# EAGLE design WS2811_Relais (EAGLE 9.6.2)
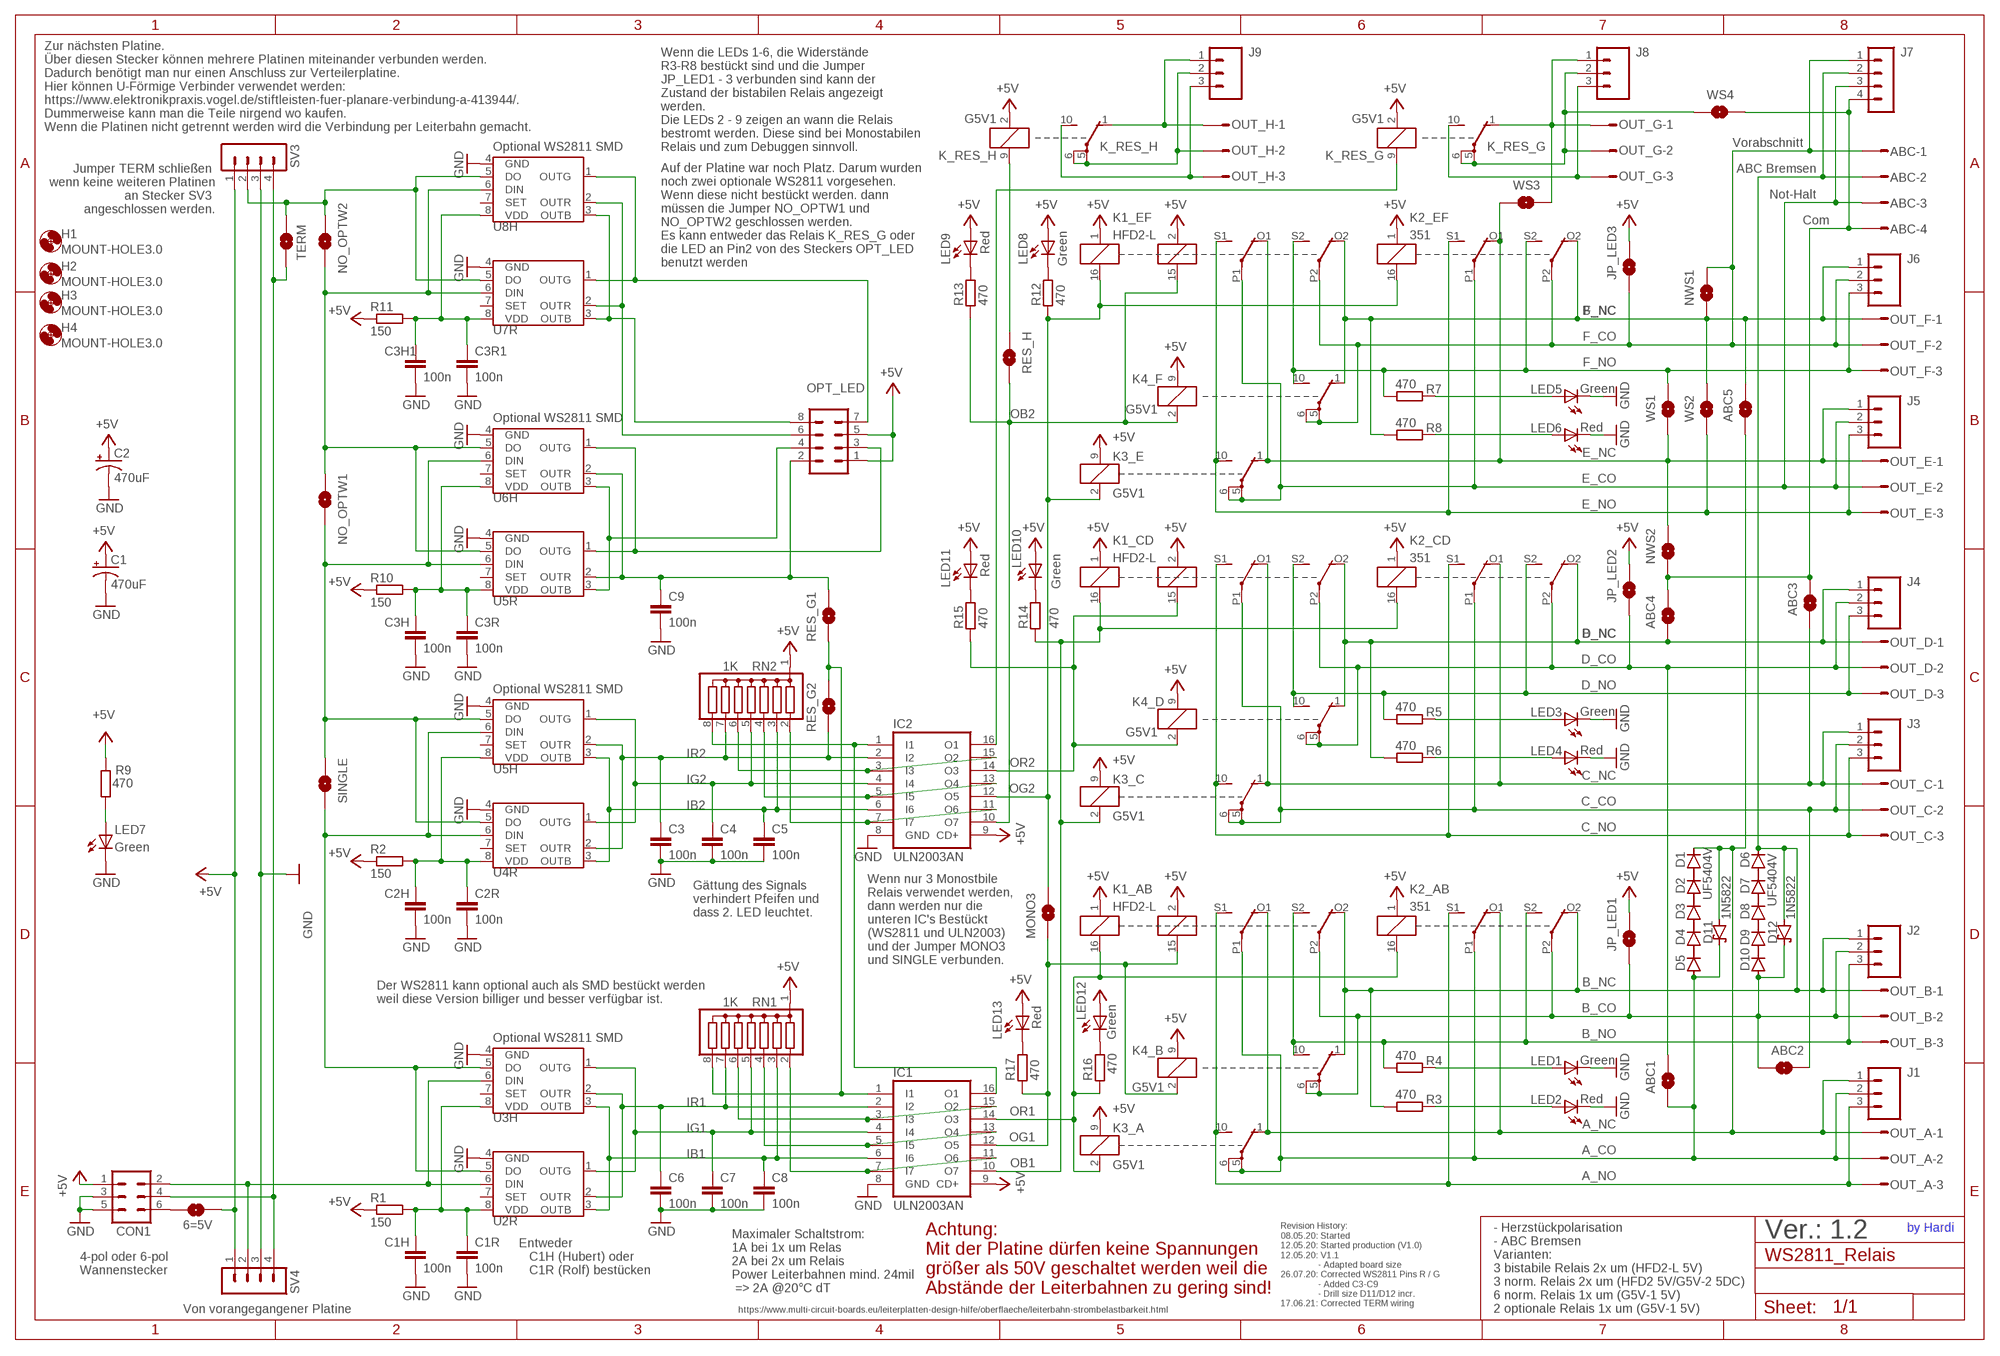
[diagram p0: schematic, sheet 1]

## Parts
6=5V  SOLDERJUMPERNO  [SJ_2S-NO]
ABC  STL1550-4ON_BOARD  [STL1550-4_ON_BOARD]
ABC1  SOLDERJUMPERNO  [SJ_2S-NO]
ABC2  SOLDERJUMPERNO  [SJ_2S-NO]
ABC3  SOLDERJUMPERNO  [SJ_2S-NO]
ABC4  SOLDERJUMPERNO  [SJ_2S-NO]
ABC5  SOLDERJUMPERNO  [SJ_2S-NO]
C1  470uF  SPARKFUN-CAPACITORS_100UF-25V-20%(PTH)  [SPARKFUN-CAPACITORS_CPOL-RADIAL-100UF-25V]
C1H  100n  C-EUC1206  [C1206]
C1R  100n  C-EU025-024X044  [C025-024X044]
C2  470uF  SPARKFUN-CAPACITORS_100UF-25V-20%(PTH)  [SPARKFUN-CAPACITORS_CPOL-RADIAL-100UF-25V]
C2H  100n  C-EUC1206  [C1206]
C2R  100n  C-EU025-024X044  [C025-024X044]
C3  100n  C-EU025-024X044  [C025-024X044]
C3H  100n  C-EUC1206  [C1206]
C3H1  100n  C-EUC1206  [C1206]
C3R  100n  C-EU025-024X044  [C025-024X044]
C3R1  100n  C-EU025-024X044  [C025-024X044]
C4  100n  C-EU025-024X044  [C025-024X044]
C5  100n  C-EU025-024X044  [C025-024X044]
C6  100n  C-EU025-024X044  [C025-024X044]
C7  100n  C-EU025-024X044  [C025-024X044]
C8  100n  C-EU025-024X044  [C025-024X044]
C9  100n  C-EU025-024X044  [C025-024X044]
CON1  ML6  [ML6]
D1  UF5404V  [DO201-15-V]
D2  UF5404V  [DO201-15-V]
D3  UF5404V  [DO201-15-V]
D4  UF5404V  [DO201-15-V]
D5  UF5404V  [DO201-15-V]
D6  UF5404V  [DO201-15-V]
D7  UF5404V  [DO201-15-V]
D8  UF5404V  [DO201-15-V]
D9  UF5404V  [DO201-15-V]
D10  UF5404V  [DO201-15-V]
D11  1N5822  [DO41-7.6]
D12  1N5822  [DO41-7.6]
H1  MOUNT-HOLE3.0  [3,0]
H2  MOUNT-HOLE3.0  [3,0]
H3  MOUNT-HOLE3.0  [3,0]
H4  MOUNT-HOLE3.0  [3,0]
IC1  ULN2003AN  [DIL16]
IC2  ULN2003AN  [DIL16]
J1  M03PTH  [1X03]
J2  M03PTH  [1X03]
J3  M03PTH  [1X03]
J4  M03PTH  [1X03]
J5  M03PTH  [1X03]
J6  M03PTH  [1X03]
J7  MA04-1  [MA04-1]
J8  M03PTH  [1X03]
J9  M03PTH  [1X03]
JP_LED1  SOLDERJUMPERNO  [SJ_2S-NO]
JP_LED2  SOLDERJUMPERNO  [SJ_2S-NO]
JP_LED3  SOLDERJUMPERNO  [SJ_2S-NO]
K1_AB  HFD2-L  [HFD2-L]
K1_CD  HFD2-L  [HFD2-L]
K1_EF  HFD2-L  [HFD2-L]
K2_AB  351  [351]
K2_CD  351  [351]
K2_EF  351  [351]
K3_A  G5V1  [G5V1]
K3_C  G5V1  [G5V1]
K3_E  G5V1  [G5V1]
K4_B  G5V1  [G5V1]
K4_D  G5V1  [G5V1]
K4_F  G5V1  [G5V1]
K_RES_G  G5V1  [G5V1]
K_RES_H  G5V1  [G5V1]
LED1  Green  LED3MM  [LED3MM]
LED2  Red  LED3MM  [LED3MM]
LED3  Green  LED3MM  [LED3MM]
LED4  Red  LED3MM  [LED3MM]
LED5  Green  LED3MM  [LED3MM]
LED6  Red  LED3MM  [LED3MM]
LED7  Green  LED3MM  [LED3MM]
LED8  Green  LED3MM  [LED3MM]
LED9  Red  LED3MM  [LED3MM]
LED10  Green  LED3MM  [LED3MM]
LED11  Red  LED3MM  [LED3MM]
LED12  Green  LED3MM  [LED3MM]
LED13  Red  LED3MM  [LED3MM]
MONO3  SOLDERJUMPERNO  [SJ_2S-NO]
NO_OPTW1  SOLDERJUMPERNO  [SJ_2S-NO]
NO_OPTW2  SOLDERJUMPERNO  [SJ_2S-NO]
NWS1  SOLDERJUMPERNO  [SJ_2S-NO]
NWS2  SOLDERJUMPERNO  [SJ_2S-NO]
OPT_LED  CON-HARTING-ML_ML08  [CON-HARTING-ML_ML08]
OUT_A  STL1550-3  [STL1550-3]
OUT_B  STL1550-3  [STL1550-3]
OUT_C  STL1550-3  [STL1550-3]
OUT_D  STL1550-3  [STL1550-3]
OUT_E  STL1550-3  [STL1550-3]
OUT_F  STL1550-3  [STL1550-3]
OUT_G  STL1550-3  [STL1550-3]
OUT_H  STL1550-3  [STL1550-3]
R1  150  RCL_R-EU_0207/2V  [RCL_0207/2V]
R2  150  RCL_R-EU_0207/2V  [RCL_0207/2V]
R3  470  R0204/2V  [0204/2V]
R4  470  R0204/2V  [0204/2V]
R5  470  R0204/2V  [0204/2V]
R6  470  R0204/2V  [0204/2V]
R7  470  R0204/2V  [0204/2V]
R8  470  R0204/2V  [0204/2V]
R9  470  R0204/2V  [0204/2V]
R10  150  RCL_R-EU_0207/2V  [RCL_0207/2V]
R11  150  RCL_R-EU_0207/2V  [RCL_0207/2V]
R12  470  R0204/2V  [0204/2V]
R13  470  R0204/2V  [0204/2V]
R14  470  R0204/2V  [0204/2V]
R15  470  R0204/2V  [0204/2V]
R16  470  R0204/2V  [0204/2V]
R17  470  R0204/2V  [0204/2V]
RES_G1  SOLDERJUMPERNO  [SJ_2S-NO]
RES_G2  SOLDERJUMPERNO  [SJ_2S-NO]
RES_H  SOLDERJUMPERNO  [SJ_2S-NO]
RN1  1K  G07R  [SIL8]
RN2  1K  G07R  [SIL8]
SINGLE  SOLDERJUMPERNO  [SJ_2S-NO]
SV3  MA04-1  [MA04-1]
SV4  MA04-1  [MA04-1]
TERM  SOLDERJUMPERNO  [SJ_2S-NO]
U2R  TINY45-20-DIP  S3PO_MODUL_WS2811_SOUND_MP3-TF-16P_WS2811_AND_ATTINY_WS2811-ICTINY45-20-DIP  [S3PO_MODUL_WS2811_SOUND_MP3-TF-16P_WS2811_AND_ATTINY_WS2811_DIP08]
U3H  WS2811 SOT-8  S3PO_MODUL_WS2811_SOUND_MP3-TF-16P_WS2811_AND_ATTINY_WS2811-ICSOP8  [SOP8]
U4R  TINY45-20-DIP  S3PO_MODUL_WS2811_SOUND_MP3-TF-16P_WS2811_AND_ATTINY_WS2811-ICTINY45-20-DIP  [S3PO_MODUL_WS2811_SOUND_MP3-TF-16P_WS2811_AND_ATTINY_WS2811_DIP08]
U5H  WS2811 SOT-8  S3PO_MODUL_WS2811_SOUND_MP3-TF-16P_WS2811_AND_ATTINY_WS2811-ICSOP8  [SOP8]
U5R  TINY45-20-DIP  S3PO_MODUL_WS2811_SOUND_MP3-TF-16P_WS2811_AND_ATTINY_WS2811-ICTINY45-20-DIP  [S3PO_MODUL_WS2811_SOUND_MP3-TF-16P_WS2811_AND_ATTINY_WS2811_DIP08]
U6H  WS2811 SOT-8  S3PO_MODUL_WS2811_SOUND_MP3-TF-16P_WS2811_AND_ATTINY_WS2811-ICSOP8  [SOP8]
U7R  TINY45-20-DIP  S3PO_MODUL_WS2811_SOUND_MP3-TF-16P_WS2811_AND_ATTINY_WS2811-ICTINY45-20-DIP  [S3PO_MODUL_WS2811_SOUND_MP3-TF-16P_WS2811_AND_ATTINY_WS2811_DIP08]
U8H  WS2811 SOT-8  S3PO_MODUL_WS2811_SOUND_MP3-TF-16P_WS2811_AND_ATTINY_WS2811-ICSOP8  [SOP8]
WS1  SOLDERJUMPERNO  [SJ_2S-NO]
WS2  SOLDERJUMPERNO  [SJ_2S-NO]
WS3  SOLDERJUMPERNO  [SJ_2S-NO]
WS4  SOLDERJUMPERNO  [SJ_2S-NO]

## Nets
+5V: 6=5V.2 C1.1(+) C2.1(+) CON1.1 IC1.9(CD+) IC2.9(CD+) JP_LED1.2 JP_LED2.2 JP_LED3.2 K1_AB.1 K1_AB.2 K1_CD.1 K1_CD.2 K1_EF.1 K1_EF.2 K2_AB.1 K2_CD.1 K2_EF.1 K3_A.9 K3_C.9 K3_E.9 K4_B.9 K4_D.9 K4_F.9 K_RES_G.2 K_RES_H.2 LED8.A LED9.A LED10.A LED11.A LED12.A LED13.A OPT_LED.1 OPT_LED.5 R1.1 R2.1 R9.1 R10.1 R11.1 RN1.1 RN2.1 SV3.1 SV4.1
A_CO: ABC1.1 D5.A D11.C J1.2 K1_AB.P1(2:P) K2_AB.P1(2:P) K3_A.5(2:P) K3_A.6(2:P) OUT_A.2
A_NC: ABC5.2 D1.C D11.A J1.1 K1_AB.O1(2:O) K2_AB.O1(2:O) K3_A.1(2:O) OUT_A.1
A_NO: J1.3 K1_AB.S1(2:S) K2_AB.S1(2:S) K3_A.10(2:S) OUT_A.3
B_CO: ABC2.1 D10.A D12.C J2.2 JP_LED1.1 K1_AB.P2(3:P) K2_AB.P2(3:P) K4_B.5(2:P) K4_B.6(2:P) OUT_B.2
B_NC: ABC.2 D6.C D12.A J2.1 J7.2 K1_AB.O2(3:O) K2_AB.O2(3:O) K4_B.1(2:O) OUT_B.1 R3.2
B_NO: J2.3 K1_AB.S2(3:S) K2_AB.S2(3:S) K4_B.10(2:S) OUT_B.3 R4.2
C_CO: ABC2.2 J3.2 K1_CD.P1(2:P) K2_CD.P1(2:P) K3_C.5(2:P) K3_C.6(2:P) OUT_C.2
C_NC: ABC3.2 J3.1 K1_CD.O1(2:O) K2_CD.O1(2:O) K3_C.1(2:O) OUT_C.1
C_NO: J3.3 K1_CD.S1(2:S) K2_CD.S1(2:S) K3_C.10(2:S) OUT_C.3
COM: ABC3.1 ABC4.1 ABC.4 J7.4 NWS2.2 WS4.1
CTRL_H_OB2: K_RES_H.9 RES_H.2
D_CO: ABC1.2 J4.2 JP_LED2.1 K1_CD.P2(3:P) K2_CD.P2(3:P) K4_D.5(2:P) K4_D.6(2:P) OUT_D.2
D_NC: ABC4.2 J4.1 K1_CD.O2(3:O) K2_CD.O2(3:O) K4_D.1(2:O) OUT_D.1 R6.2
D_NO: J4.3 K1_CD.S2(3:S) K2_CD.S2(3:S) K4_D.10(2:S) OUT_D.3 R5.2
DI_WS1: CON1.2 SV4.2 U2R.6(DIN) U3H.6(DIN)
DO1_DI2: SINGLE.2 U2R.5(DO) U3H.5(DO) U4R.6(DIN) U5H.6(DIN)
DO2_DI3: NO_OPTW1.2 SINGLE.1 U4R.5(DO) U5H.5(DO) U5R.6(DIN) U6H.6(DIN)
DO3_DI4: NO_OPTW1.1 NO_OPTW2.2 U5R.5(DO) U6H.5(DO) U7R.6(DIN) U8H.6(DIN)
DO4_NEXT_TERM: NO_OPTW2.1 SV3.2 TERM.2 U7R.5(DO) U8H.5(DO)
DO_RETURN: CON1.4 SV3.4 SV4.4 TERM.1
E_CO: ABC.3 J5.2 J7.3 K1_EF.P1(2:P) K2_EF.P1(2:P) K3_E.5(2:P) K3_E.6(2:P) OUT_E.2
E_NC: J5.1 K1_EF.O1(2:O) K2_EF.O1(2:O) K3_E.1(2:O) NWS2.1 OUT_E.1 WS1.2 WS3.2
E_NO: J5.3 K1_EF.S1(2:S) K2_EF.S1(2:S) K3_E.10(2:S) OUT_E.3 WS2.2
F_CO: ABC.1 J6.2 J7.1 JP_LED3.1 K1_EF.P2(3:P) K2_EF.P2(3:P) K4_F.5(2:P) K4_F.6(2:P) NWS1.1 OUT_F.2
F_NC: ABC5.1 J6.1 K1_EF.O2(3:O) K2_EF.O2(3:O) K4_F.1(2:O) NWS1.2 OUT_F.1 R8.2 WS2.1
F_NO: J6.3 K1_EF.S2(3:S) K2_EF.S2(3:S) K4_F.10(2:S) OUT_F.3 R7.2 WS1.1
G_COM: J8.2 K_RES_G.5(2:P) K_RES_G.6(2:P) OUT_G.2 WS4.2
G_NC: J8.1 K_RES_G.1(2:O) OUT_G.1 WS3.1
G_NO: J8.3 K_RES_G.10(2:S) OUT_G.3
GND: C1.2(-) C1H.2 C1R.2 C2.2(-) C2H.2 C2R.2 C3.2 C3H1.2 C3H.2 C3R1.2 C3R.2 C4.2 C5.2 C6.2 C7.2 C8.2 C9.2 CON1.3 CON1.5 IC1.8(GND) IC2.8(GND) LED1.K(C) LED2.K(C) LED3.K(C) LED4.K(C) LED5.K(C) LED6.K(C) LED7.K(C) SV3.3 SV4.3 U2R.4(GND) U3H.4(GND) U4R.4(GND) U5H.4(GND) U5R.4(GND) U6H.4(GND) U7R.4(GND) U8H.4(GND)
H_COM: J9.2 K_RES_H.5(2:P) K_RES_H.6(2:P) OUT_H.2
H_NC: J9.1 K_RES_H.1(2:O) OUT_H.1
H_NO: J9.3 K_RES_H.10(2:S) OUT_H.3
IB1: C8.1 IC1.6(I6) RN1.3 U2R.3(OUTB) U3H.3(OUTB)
IB1_2: IC1.7(I7) IC1.11(O6) RN1.2
IB2: C5.1 IC2.6(I6) RN2.3 U4R.3(OUTB) U5H.3(OUTB)
IB2_2: IC2.7(I7) IC2.11(O6) RN2.2
IB3: OPT_LED.4 U5R.3(OUTB) U6H.3(OUTB)
IB4: OPT_LED.8 U7R.3(OUTB) U8H.3(OUTB)
IG1: C7.1 IC1.4(I4) RN1.5 U2R.1(OUTG) U3H.1(OUTG)
IG1_2: IC1.5(I5) IC1.13(O4) RN1.4
IG2: C4.1 IC2.4(I4) RN2.5 U4R.1(OUTG) U5H.1(OUTG)
IG2_2: IC2.5(I5) IC2.13(O4) RN2.4
IG3: OPT_LED.3 U5R.1(OUTG) U6H.1(OUTG)
IG4: OPT_LED.7 U7R.1(OUTG) U8H.1(OUTG)
IR1: C6.1 IC1.2(I2) RN1.7 U2R.2(OUTR) U3H.2(OUTR)
IR1_2: IC1.3(I3) IC1.15(O2) RN1.6
IR2: C3.1 IC2.2(I2) RES_G2.2 RN2.7 U4R.2(OUTR) U5H.2(OUTR)
IR2_2: IC2.3(I3) IC2.15(O2) RN2.6
IR3: IC1.1(I1) RES_G1.2 RES_G2.1 RN1.8
IR3_2: C9.1 OPT_LED.2 RES_G1.1 U5R.2(OUTR) U6H.2(OUTR)
IR3_3: IC1.16(O1) IC2.1(I1) RN2.8
IR4: OPT_LED.6 U7R.2(OUTR) U8H.2(OUTR)
LED2: LED2.A R3.1
LED3: LED3.A R5.1
LED4: LED4.A R6.1
LED_1: LED1.A R4.1
LED_5: LED5.A R7.1
LED_6: LED6.A R8.1
LED_7: LED7.A R9.2
N$6: 6=5V.1 CON1.6
N$16: D1.A D2.C
N$19: D2.A D3.C
N$21: D3.A D4.C
N$23: D4.A D5.C
N$24: D7.A D8.C
N$25: D8.A D9.C
N$26: D9.A D10.C
N$27: D6.A D7.C
N$42: LED8.K(C) R12.1
N$43: LED9.K(C) R13.1
N$44: LED10.K(C) R14.1
N$45: LED11.K(C) R15.1
N$46: LED12.K(C) R16.1
N$47: LED13.K(C) R17.1
OB1: IC1.10(O7) K1_CD.16 K2_CD.16 K3_C.2 R14.2
OB2: IC2.10(O7) K1_EF.15 K4_F.2 R13.2 RES_H.1
OG1: IC1.12(O5) K1_AB.15 K4_B.2 MONO3.2 R17.2
OG2: IC2.12(O5) K1_EF.16 K2_EF.16 K3_E.2 MONO3.1 R12.2
OR1: IC1.14(O3) K1_AB.16 K2_AB.16 K3_A.2 R16.2
OR2: IC2.14(O3) K1_CD.15 K4_D.2 R15.2
OR3: IC2.16(O1) K_RES_G.9
PWR_WS1: C1H.1 C1R.1 R1.2 U2R.8(VDD) U3H.8(VDD)
PWR_WS2: C2H.1 C2R.1 R2.2 U4R.8(VDD) U5H.8(VDD)
PWR_WS3: C3H.1 C3R.1 R10.2 U5R.8(VDD) U6H.8(VDD)
PWR_WS4: C3H1.1 C3R1.1 R11.2 U7R.8(VDD) U8H.8(VDD)
Unconnected: U2R.7(SET) U3H.7(SET) U4R.7(SET) U5H.7(SET) U5R.7(SET) U6H.7(SET) U7R.7(SET) U8H.7(SET)

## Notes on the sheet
- Wenn die LEDs 1-6, die Widerstände
  R3-R8 bestückt sind und die Jumper 
  JP_LED1 - 3 verbunden sind kann der 
  Zustand der bistabilen Relais angezeigt
  werden. 
  Die LEDs 2 - 9 zeigen an wann die Relais
  bestromt werden. Diese sind bei Monostabilen
  Relais und zum Debuggen sinnvoll.
- Zur nächsten Platine. 
  Über diesen Stecker können mehrere Platinen miteinander verbunden werden.
  Dadurch benötigt man nur einen Anschluss zur Verteilerplatine.
  Hier können U-Förmige Verbinder verwendet werden: 
  https://www.elektronikpraxis.vogel.de/stiftleisten-fuer-planare-verbindung-a-413944/.
  Dummerweise kann man die Teile nirgend wo kaufen.
  Wenn die Platinen nicht getrennt werden wird die Verbindung per Leiterbahn gemacht.
- Vorabschnitt
- Optional WS2811 SMD
- Jumper TERM schließen 
  wenn keine weiteren Platinen
  an Stecker SV3 
  angeschlossen werden.
- ABC Bremsen
- Not-Halt
- Com
- Auf der Platine war noch Platz. Darum wurden
  noch zwei optionale WS2811 vorgesehen. 
  Wenn diese nicht bestückt werden. dann 
  müssen die Jumper NO_OPTW1 und 
  NO_OPTW2 geschlossen werden. 
  Es kann entweder das Relais K_RES_G oder 
  die LED an Pin2 von des Steckers OPT_LED 
  benutzt werden
- Optional WS2811 SMD
- Optional WS2811 SMD
- Gättung des Signals
  verhindert Pfeifen und
  dass 2. LED leuchtet.
- Wenn nur 3 Monostbile
  Relais verwendet werden,
  dann werden nur die
  unteren IC's Bestückt
  (WS2811 und ULN2003)
  und der Jumper MONO3
  und SINGLE verbunden.
- Der WS2811 kann optional auch als SMD bestückt werden
  weil diese Version billiger und besser verfügbar ist.
- Optional WS2811 SMD
- Ver.: 1.2
- Achtung:
  Mit der Platine dürfen keine Spannungen
  größer als 50V geschaltet werden weil die
  Abstände der Leiterbahnen zu gering sind!
- Revision History:
  08.05.20: Started
  12.05.20: Started production (V1.0)
  12.05.20: V1.1
                 - Adapted board size
  26.07.20: Corrected WS2811 Pins R / G
                 - Added C3-C9
                 - Drill size D11/D12 incr.
  17.06.21: Corrected TERM wiring
- - Herzstückpolarisation
  - ABC Bremsen
  Varianten:
  3 bistabile Relais 2x um (HFD2-L 5V)
  3 norm. Relais 2x um (HFD2 5V/G5V-2 5DC)
  6 norm. Relais 1x um (G5V-1 5V)
  2 optionale Relais 1x um (G5V-1 5V)
- by Hardi
- Maximaler Schaltstrom:
  1A bei 1x um Relas
  2A bei 2x um Relais
  Power Leiterbahnen mind. 24mil
   => 2A @20°C dT
- 4-pol oder 6-pol 
  Wannenstecker
- Entweder 
     C1H (Hubert) oder 
     C1R (Rolf) bestücken
- https://www.multi-circuit-boards.eu/leiterplatten-design-hilfe/oberflaeche/leiterbahn-strombelastbarkeit.html
- Von vorangegangener Platine

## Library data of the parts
6=5V ABC1-ABC5 JP_LED1-JP_LED3 MONO3 NO_OPTW1 NO_OPTW2 NWS1 NWS2 RES_G1 RES_G2 RES_H SINGLE TERM WS1-WS4 = SparkFun-Retired:SOLDERJUMPER: Solder Jumper
ABC = SchraubStecker3.5:STL1550-4: CONNECTOR Rastermass 3.5 mm Kabel: AK(Z)1550 Platine: STL(Z)1550 Ali: KF2EDG-3.5
C1 C2 = Sound_MP3-TF-16P_and_WS2811:SPARKFUN-CAPACITORS_100UF-25V-20%(PTH): CAP-08439; PROD_ID: CAP-08439
C1H C1R C2H C2R C3 C3H C3H1 C3R C3R1 C4-C9 = rcl:C-EU: CAPACITOR, European symbol; SPICEPREFIX: C
CON1 = con-harting-ml:ML6: HARTING; OC_FARNELL: unknown; OC_NEWARK: unknown
D1-D10 = diode:UF5404: DIODE
D11 D12 = diode:1N5822: 1.0A SCHOTTKY BARRIER RECTIFIER
H1-H4 = holes:MOUNT-HOLE: MOUNTING HOLE with drill center marker
IC1 IC2 = uln-udn:ULN2003A: DRIVER ARRAY; REICHELT: ULN 2003A STM; REICHELT_EU: 0,22 €; REICHELT_LNK: https://www.reichelt.de/seven-darlington-arrays-dip-16-uln-2003a-stm-p216685.html?&trstct=pos_0
J1-J6 J8 J9 = SparkFun-Connectors:M03: Header 3 Standard 3-pin 0.1" header. Use with straight break away headers (SKU : PRT-00116), right angle break away headers (PRT-00553), swiss pins (PRT-00743), machine pins (PRT-00117), and female headers (PRT-00115). Molex polarized connector foot print use with SKU : PRT-08232 with associated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
J7 SV3 SV4 = con-lstb:MA04-1: PIN HEADER
K1_AB K1_CD K1_EF = WS2811_Relais:HFD2-L: RELAY 2 x switch, HFD2-L by Hardi; OC_FARNELL: unknown; OC_NEWARK: unknown
K2_AB K2_CD K2_EF = relay:351: RELAY 2 x switch, Omron; OC_FARNELL: unknown; OC_NEWARK: unknown
K3_A K3_C K3_E K4_B K4_D K4_F K_RES_G K_RES_H = relay:G5V1: RELAY 1 x switch, 0.5 A/125 V AC, 1 A/24 V DC , Omron; MPN: G5V-1-DC24; OC_FARNELL: 9949593; OC_NEWARK: 36M6377
LED1-LED13 = Arduino_fuer_LEDs_DCC_2:LED: LED
OPT_LED = PushButtonAction_4017_2:CON-HARTING-ML_ML08: Modified by Hardi; OC_FARNELL: unknown; OC_NEWARK: unknown
OUT_A OUT_B OUT_C OUT_D OUT_E OUT_F OUT_G OUT_H = SchraubStecker3.5:STL1550-3: CONNECTOR Rastermass 3.5 mm Kabel: AK(Z)1550 Platine: STL(Z)1550 Ali: KF2EDG-3.5
R1 R2 R10 R11 = Sound_MP3-TF-16P_and_WS2811:RCL_R-EU_: RESISTOR, European symbol; SPICEPREFIX: R
R3-R9 R12-R17 = Arduino_fuer_LEDs_DCC_2:R: RESISTOR, European symbol
RN1 RN2 = resistor-sil:G07R: SIL RESISTOR; OC_FARNELL: unknown; OC_NEWARK: unknown
U2R U4R U5R U7R = S3PO_Modul_WS2811:S3PO_MODUL_WS2811_SOUND_MP3-TF-16P_WS2811_AND_ATTINY_WS2811-IC: Die Pin Nummern für R und G sind getauscht damit sie gleich angesteuert werden wie die WS2812. Der Daten Strom der WS2811 ist RGB, Beim WS2812 ist es aber GRB.; PROD_ID: IC-09439
U3H U5H U6H U8H = S3PO_Modul_WS2811:S3PO_MODUL_WS2811_SOUND_MP3-TF-16P_WS2811_AND_ATTINY_WS2811-IC: Die Pin Nummern für R und G sind getauscht damit sie gleich angesteuert werden wie die WS2812. Der Daten Strom der WS2811 ist RGB, Beim WS2812 ist es aber GRB.

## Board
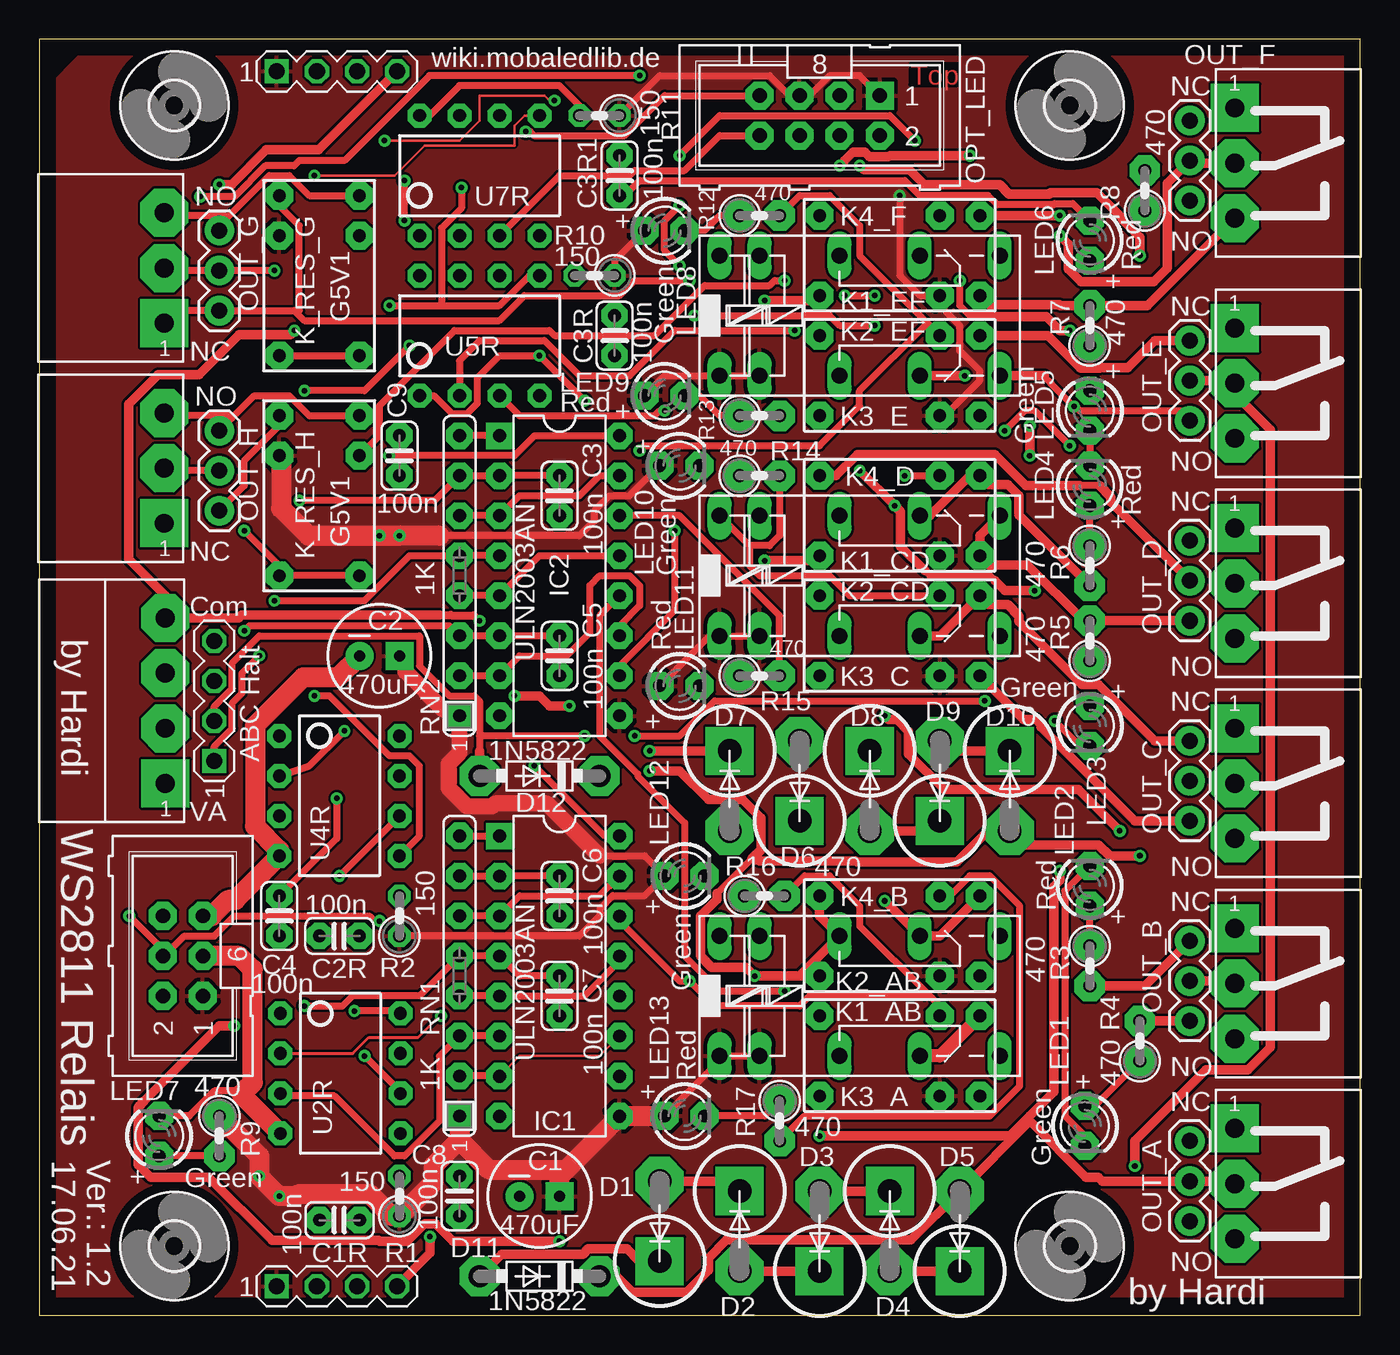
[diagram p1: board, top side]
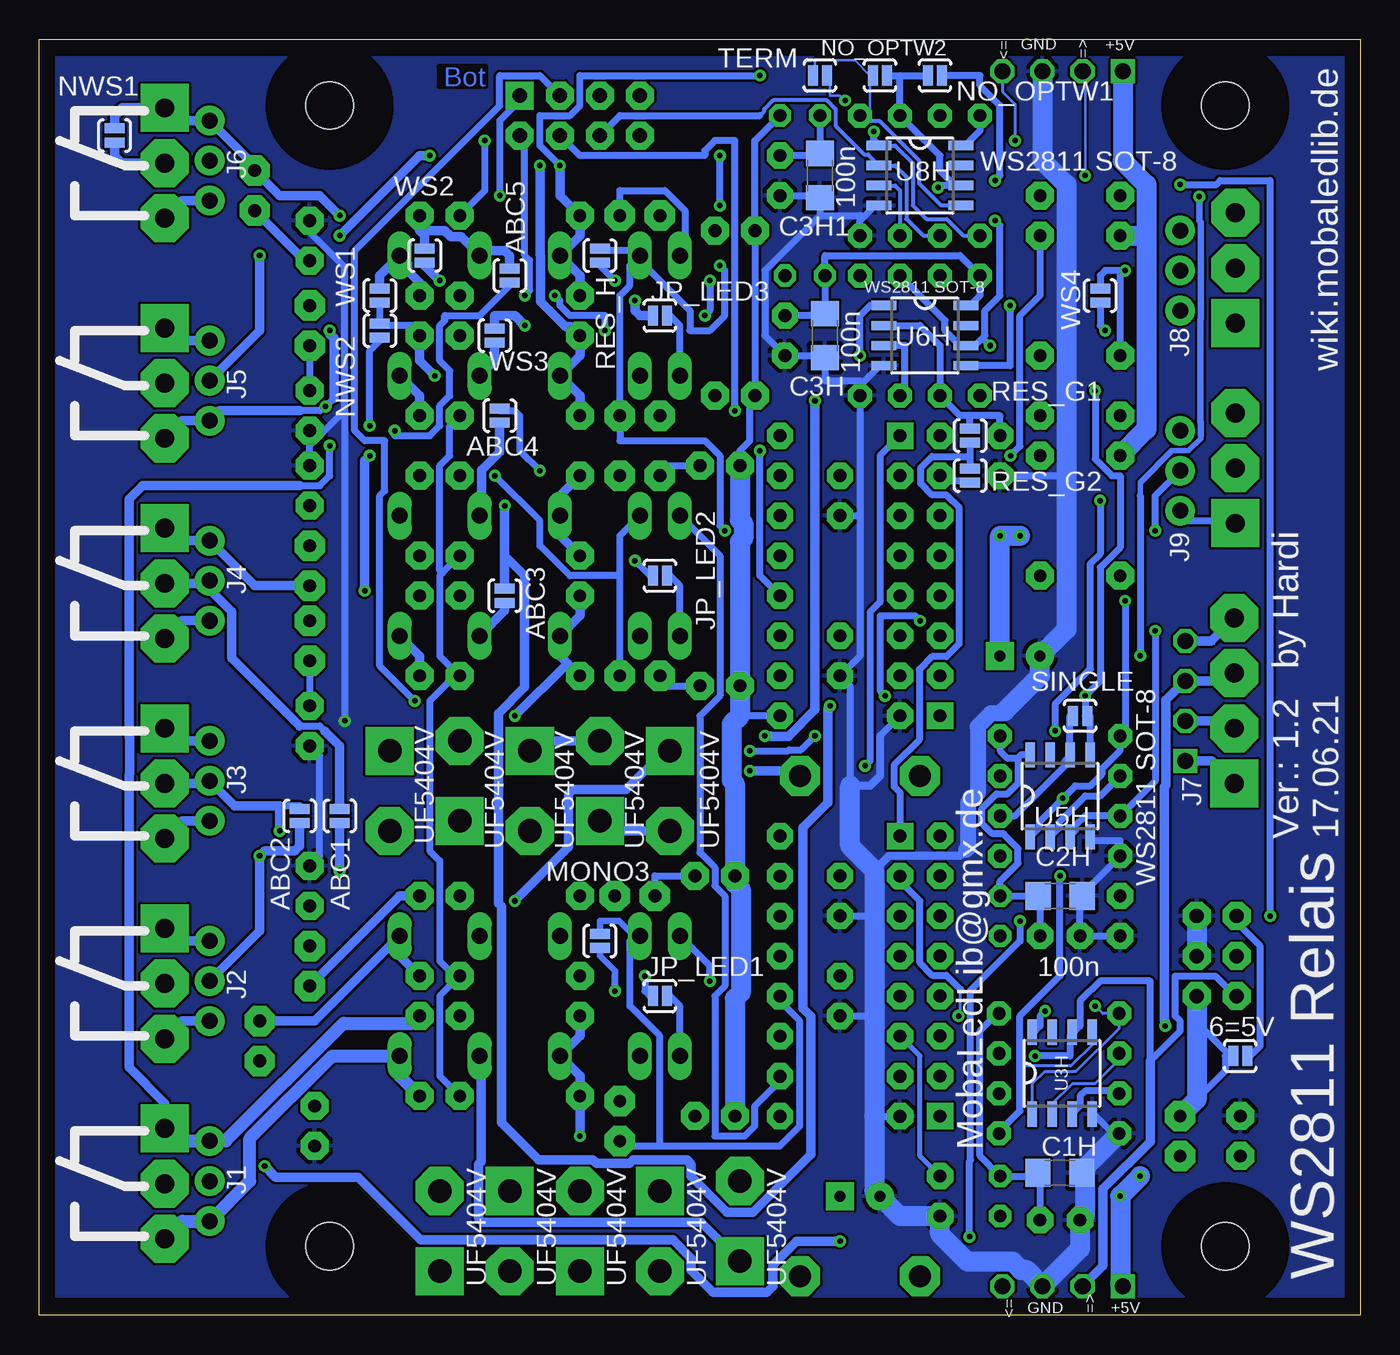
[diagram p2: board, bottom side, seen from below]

Size 83.82 x 80.97 mm. Coordinates in mm from the lower left corner, seen from the top.
Outline: 0,0 83.82,0 83.82,80.97 0,80.97 0,0
Copper layers (1*16): Top 0.035mm / dielectric 1.5mm / Bottom 0.035mm
Design rules "default *": minimum track width 6mil, minimum drill 0.35mm, track to track 6mil, track to pad 6mil, pad to pad 6mil, via to via 6mil, smd to smd 6mil, copper to edge 40mil, drill to drill 6mil, minimum pad ring 10mil, minimum via ring 8mil, stop-mask expansion 4mil, vias tented up to drill 16mil, thermal gap 10mil

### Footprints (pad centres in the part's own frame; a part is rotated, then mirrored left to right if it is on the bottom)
SJ_2S-NO = smd 0.635 x 1.27: 1 -0.45,0; 2 0.45,0
STL1550-4_ON_BOARD = drill 1.2 pad 3.048 square: 1 -1.75,0 | drill 1.2 pad 3.048 octagon: 2 1.75,0; 3 5.25,0; 4 8.75,0
SPARKFUN-CAPACITORS_CPOL-RADIAL-100UF-25V = drill 0.7 pad 1.778 square: 1 1.27,0 | drill 0.7 pad 1.778: 2 -1.27,0
C1206 = smd 1.6 x 1.8: 1 -1.4,0; 2 1.4,0
C025-024X044 = drill 0.813 pad 1.676 octagon: 1 -1.27,0; 2 1.27,0
ML6 = drill 0.914 pad 1.778 octagon: 1 -2.54,-1.27; 2 -2.54,1.27; 3 0,-1.27; 4 0,1.27; 5 2.54,-1.27; 6 2.54,1.27
DO201-15-V = drill 1.499 pad 3.048 octagon: A 5.08,0 | drill 1.499 pad 3.048 square: C 0,0
DO41-7.6 = drill 1.4 pad 2.54 octagon: A 3.81,0; C -3.81,0
3,0 = hole 3: 0,0
DIL16 = drill 0.813 pad 1.676 square: 1 -8.89,-3.81 | drill 0.813 pad 1.676 octagon: 2 -6.35,-3.81; 3 -3.81,-3.81; 4 -1.27,-3.81; 5 1.27,-3.81; 6 3.81,-3.81; 7 6.35,-3.81; 8 8.89,-3.81; 9 8.89,3.81; 10 6.35,3.81; 11 3.81,3.81; 12 1.27,3.81; 13 -1.27,3.81; 14 -3.81,3.81; 15 -6.35,3.81; 16 -8.89,3.81
1X03 = drill 1.016 pad 1.88: 1 0,0; 2 2.54,0; 3 5.08,0
MA04-1 = drill 1.016 pad 1.524 square: 1 -3.81,0 | drill 1.016 pad 1.524 octagon: 2 -1.27,0; 3 1.27,0; 4 3.81,0
HFD2-L = drill 1.016 long: 1 -3.81,-3.81; 2 -1.27,-3.81; 15 -1.27,3.81; 16 -3.81,3.81; O1 8.89,-3.81; O2 8.89,3.81; P1 3.81,-3.81; P2 3.81,3.81; S1 13.97,-3.81; S2 13.97,3.81
351 = drill 1.016 long: 1 -3.81,-3.81; 16 -3.81,3.81; O1 8.89,-3.81; O2 8.89,3.81; P1 3.81,-3.81; P2 3.81,3.81; S1 13.97,-3.81; S2 13.97,3.81
G5V1 = drill 0.813 pad 1.778 octagon: 1 -5.08,-2.54; 2 -2.54,-2.54; 5 5.08,-2.54; 6 5.08,2.54; 9 -2.54,2.54; 10 -5.08,2.54
LED3MM = drill 0.813 pad 1.778 octagon: A -1.27,0; K 1.27,0
CON-HARTING-ML_ML08 = drill 0.914 pad 1.778 square: 1 -5.08,-1.27 | drill 0.914 pad 1.778 octagon: 2 -5.08,1.27; 3 -2.54,-1.27; 4 -2.54,1.27; 5 0,-1.27; 6 0,1.27; 7 2.54,-1.27; 8 2.54,1.27
STL1550-3 = drill 1.2 pad 3.048 square: 1 -1.75,0 | drill 1.2 pad 3.048 octagon: 2 1.75,0; 3 5.25,0
RCL_0207/2V = drill 0.813 pad 1.422 octagon: 1 -1.27,0; 2 1.27,0
0204/2V = drill 0.813 pad 1.93 octagon: 1 -1.27,0; 2 1.27,0
SIL8 = drill 0.813 pad 1.676 square: 1 -8.89,0 | drill 0.813 pad 1.676 octagon: 2 -6.35,0; 3 -3.81,0; 4 -1.27,0; 5 1.27,0; 6 3.81,0; 7 6.35,0; 8 8.89,0
S3PO_MODUL_WS2811_SOUND_MP3-TF-16P_WS2811_AND_ATTINY_WS2811_DIP08 = drill 0.813 pad 1.524 octagon: 1 -3.81,-3.81; 2 -1.27,-3.81; 3 1.27,-3.81; 4 3.81,-3.81; 5 3.81,3.81; 6 1.27,3.81; 7 -1.27,3.81; 8 -3.81,3.81
SOP8 = smd 0.6 x 1.6: 1 -1.905,-2.6; 2 -0.635,-2.6; 3 0.635,-2.6; 4 1.905,-2.6; 5 1.905,2.6; 6 0.635,2.6; 7 -0.635,2.6; 8 -1.905,2.6

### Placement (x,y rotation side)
6=5V  7.61,16.45 180 bottom
ABC  7.99,35.5 90 top
ABC1  64.76,31.68 90 bottom
ABC2  67.3,31.68 90 bottom
ABC3  54.28,45.66 270 bottom
ABC4  54.6,57.09 270 bottom
ABC5  53.96,65.98 270 bottom
C1  31.74,7.55 0 top
C1H  19.05,9.03 0 bottom
C1R  19.05,6.03 180 top
C2  21.58,41.84 0 top
C2H  19.04,26.61 0 bottom
C2R  19.04,24.06 180 top
C3  33.01,52.01 270 top
C3H  33.96,62.16 270 bottom
C3H1  34.28,72.33 270 bottom
C3R  36.5,62.16 270 top
C3R1  36.82,72.33 270 top
C4  15.23,25.33 270 top
C5  33.01,41.84 270 top
C6  33.01,26.61 270 top
C7  33.01,20.25 270 top
C8  26.66,7.55 270 top
C9  22.85,54.55 270 top
CON1  9.1,22.79 90 top
D1  39.36,3.43 90 top
D2  44.44,7.87 270 top
D3  49.52,2.79 90 top
D4  53.96,7.87 270 top
D5  58.41,2.79 90 top
D6  43.8,35.81 270 top
D7  48.25,31.37 90 top
D8  52.7,35.81 270 top
D9  57.14,31.37 90 top
D10  61.58,35.81 270 top
D11  31.74,2.48 180 top
D12  31.74,34.23 180 top
H1  8.56,76.77 0 top
H2  65.39,76.77 0 top
H3  65.39,4.38 0 top
H4  8.56,4.38 0 top
IC1  33.01,21.51 270 top
IC2  33.01,46.93 270 top
J1  73.02,11.05 270 top
J2  73.02,23.75 270 top
J3  73.02,36.45 270 top
J4  73.02,49.15 270 top
J5  73.02,61.85 270 top
J6  73.02,75.82 270 top
J7  11.1,38.99 90 top
J8  11.42,63.75 90 top
J9  11.42,51.05 90 top
JP_LED1  44.44,20.25 0 bottom
JP_LED2  44.44,46.93 0 bottom
JP_LED3  44.44,63.44 0 bottom
K1_AB  46.98,20.25 0 top
K1_CD  46.98,46.93 0 top
K1_EF  46.98,63.44 0 top
K2_AB  46.98,20.25 0 top
K2_CD  46.98,46.93 0 top
K2_EF  46.98,63.44 0 top
K3_A  54.6,16.45 180 top
K3_C  54.6,43.12 180 top
K3_E  54.6,59.62 180 top
K4_B  54.6,24.06 180 top
K4_D  54.6,50.73 180 top
K4_F  54.6,67.25 180 top
K_RES_G  17.77,65.98 270 top
K_RES_H  17.77,52.01 270 top
LED1  66.35,12 270 top
LED2  66.67,27.24 90 top
LED3  66.67,37.4 270 top
LED4  66.67,52.64 90 top
LED5  66.67,57.4 270 top
LED6  66.67,68.2 90 top
LED7  7.61,11.37 90 top
LED8  39.68,68.83 0 top
LED9  39.68,58.36 0 top
LED10  40.63,53.91 0 top
LED11  40.63,39.94 0 top
LED12  40.95,27.88 0 top
LED13  40.95,12.63 0 top
MONO3  48.25,23.75 90 bottom
NO_OPTW1  26.98,78.67 0 bottom
NO_OPTW2  30.47,78.67 0 bottom
NWS1  79.05,74.87 90 bottom
NWS2  62.22,62.48 270 bottom
OPT_LED  48.25,76.14 180 top
OUT_A  75.87,10.1 270 top
OUT_B  75.87,22.79 270 top
OUT_C  75.87,35.5 270 top
OUT_D  75.87,48.2 270 top
OUT_E  75.87,60.9 270 top
OUT_F  75.87,74.87 270 top
OUT_G  7.93,64.7 90 top
OUT_H  7.93,52.01 90 top
R1  22.85,7.55 90 top
R2  22.85,25.33 90 top
R3  66.67,22.16 270 top
R4  69.84,17.4 90 top
R5  66.67,42.8 90 top
R6  66.67,47.56 270 top
R7  66.67,62.8 90 top
R8  70.16,71.37 90 top
R9  11.42,11.37 270 top
R10  35.23,65.98 180 top
R11  35.55,76.14 180 top
R12  45.71,69.78 0 top
R13  45.71,57.09 0 top
R14  45.71,53.28 0 top
R15  45.71,40.58 0 top
R16  46.03,26.61 0 top
R17  46.98,12.32 270 top
RES_G1  24.75,55.82 270 bottom
RES_G2  24.75,53.28 270 bottom
RES_H  48.25,67.25 270 bottom
RN1  26.66,21.52 90 top
RN2  26.66,46.93 90 top
SINGLE  17.77,38.04 180 bottom
SV3  18.88,78.93 0 top
SV4  18.88,1.84 0 top
TERM  34.28,78.67 180 bottom
U2R  19.1,15.33 270 top
U3H  18.91,15.36 0 bottom
U4R  19.04,32.96 270 top
U5H  19.04,32.96 0 bottom
U5R  27.93,62.16 0 top
U6H  27.61,62.16 270 bottom
U7R  27.93,72.33 0 top
U8H  27.93,72.33 270 bottom
WS1  62.22,64.7 270 bottom
WS2  59.36,67.25 270 bottom
WS3  54.92,62.16 270 bottom
WS4  16.5,64.7 90 bottom

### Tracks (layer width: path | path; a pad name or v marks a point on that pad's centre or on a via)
+5V  (via drill 0.35)
  Top 0.457: 43.49,16.45 K1_AB.2 | 43.49,16.45 LED13.A | 43.49,16.45 K2_AB.1 | K1_CD.2 K2_CD.1 42.53,43.12 LED11.A | 35.55,29.14 38.41,29.14 LED12.A 38.41,26.61 36.38,26.61 35.6,25.83 35.6,25.39 34.28,24.06 34.24,24.1 22.89,24.1 R2.1 | K3_E.9 57.46,57.09 59.68,59.31 59.68,59.94 58.41,61.21 58.41,62.8 57.14,64.07 K4_F.9 55.87,64.7 54.6,65.98 v54.6,71.06 | K1_EF.2 K2_EF.1 39.68,59.62 LED9.A | OPT_LED.1 52.06,78.67 50.15,78.67 48.88,77.41 OPT_LED.5 47.61,77.41 46.34,78.67 39.36,78.67 R11.1 | R10.1 36.5,66.93 LED8.A | LED10.A 37.45,52.01 36.18,52.01 35.23,51.05 35.23,50.42 34.28,49.47 25.39,49.47
  Top 1.016: C2.1 23.23,41.46 23.23,40.84 25.66,38.42 26.28,38.42 RN2.1 26.66,35.69 26,35.03 26,33.43 27.13,32.3 28.73,32.3 28.91,32.47 32.22,32.47 35.55,29.14
  Top 1.27: LED13.A 39.66,12.62 IC1.9 33.43,9.23 | R9.1 13.96,10.1 v13.96,8.83 v15.23,7.55 16.3,7.55 16.4,7.66 20.99,7.66 22.36,6.28 R1.1 25.03,8.47 25.03,9.5 26.66,11.12 | K_RES_H.2 15.33,54.44 15.33,51.21 17.07,49.47 v21.58,49.47 v22.85,49.47 25.39,49.47 | RN1.1 26.66,11.12 | 26.66,11.12 28.55,9.23 33.43,9.23 | C1.1 33.01,8.81 33.43,9.23
  Bottom 0.457: 8.4,16.6 10.15,18.35 10.15,20.25 CON1.1 | 8.4,16.6 8.25,16.45 6=5V.2 | R9.1 8.56,15.49 8.56,16.45 8.4,16.6 | K2_AB.1 43.17,19.62 43.8,20.25 JP_LED1.2 | K2_CD.1 43.17,46.29 43.8,46.93 JP_LED2.2 | IC2.9 39.36,38.04 | LED12.A LED13.A | K3_A.9 58.41,15.18 58.41,20.25 K4_B.9 57.46,21.52 58.41,22.48 58.41,28.83 59.04,29.46 59.04,38.99 57.46,40.58 K3_C.9 58.41,41.84 58.41,46.93 58.25,47.08 | K4_D.9 58.25,47.08 | K3_E.9 57.77,56.45 57.77,54.55 58.41,53.91 58.41,47.24 58.25,47.08 | K2_EF.1 43.17,62.8 43.8,63.44 JP_LED3.2 | LED10.A 39.36,54.86 38.72,55.5 38.72,58.04 LED9.A LED8.A 38.41,74.55 R11.1 | v54.6,71.06 54.6,75.82 53.33,77.09 OPT_LED.1
  Bottom 1.27: LED10.A 39.36,50.48 39.15,50.27 39.15,49.3 39.36,49.09 LED11.A 39.36,38.04 39.89,37.5 39.89,33.95 39.68,33.74 LED12.A 39.68,27.41 39.3,27.03 39.3,20.47 39.68,20.09 LED13.A | v15.23,7.55 15.23,2 SV4.1 | CON1.1 10.37,13.68 R9.1 | v13.96,8.83 15.17,7.62 | SV3.1 15.07,73.27 13.55,71.75 13.55,68.52 | K_RES_H.2 13.55,56.22 13.55,68.52 | K_RES_G.2 13.55,68.52 | C2.1 v22.85,49.47 v21.58,49.47
  pour Top: 0.62,78.04 2.53,79.95 83.81,79.95 83.81,1.21 0.62,1.21
A_CO  (via drill 0.35)
  Top 0.457: 62.85,12.32 62.85,12.63
  Top 0.61: v49.52,11.37 61.58,11.37 62.85,12.63 64.39,14.17 64.39,27.21 64.76,27.57 v64.76,28.19 | OUT_A.2 75.71,8.51 J1.2 67.45,8.51 67.2,8.75 66.42,8.75 62.85,12.32 D5.A 55.31,4.77 43.62,4.77 42.46,3.61 42.46,2.83 41.07,1.45 37.65,1.45 36.62,2.48 D11.C
  Bottom 0.61: v49.52,11.37 K3_A.6 49.52,15.18 K1_AB.P1 49.52,17.71 K3_A.5 | ABC1.1 v64.76,28.19
A_NC  (via drill 0.35)
  Top 0.457: v61.27,56.13 62.54,57.4 63.17,57.4 v65.39,55.18
  Top 0.61: D1.C 38.06,3.43 37.28,4.2 34.84,4.2 34.49,3.86 29.32,3.86 D11.A
  Top 0.813: K3_A.1 57.14,16.45 K1_AB.O1
  Bottom 0.457: v61.27,56.13 61.27,55.82 59.04,55.82 58.41,56.45 58.41,57.72 57.77,58.36 57.77,59.94 58.41,60.58 58.41,62.8 58.09,63.12 58.09,63.44 55.87,63.44 53.96,65.34 ABC5.2 | v65.39,55.18 65.39,53.28 66.03,52.64 67.3,52.64
  Bottom 0.61: OUT_A.1 75.87,13.46 78.13,15.71 78.13,34.31 78.09,34.34 78.09,36.65 78.13,36.68 78.13,51.78 77.27,52.64 67.3,52.64 | D1.C 41.82,5.89 55.68,5.89 55.95,6.16 55.95,9.59 55.79,9.74 55.79,16.37 K1_AB.O1
  Bottom 0.813: OUT_A.1 75.08,11.05 J1.1 71.98,11.05 64.5,18.53 60.14,18.53 K3_A.1
A_NO
  Bottom 0.813: OUT_A.3 74.75,5.97 J1.3 70.46,8.52 70.46,11.21 65.22,16.45 K1_AB.S1 60.95,15.18 K3_A.10
B_CO  (via drill 0.35)
  Top 0.457: K4_B.6 48.25,21.52 | 43.01,26.76 45.23,28.99 45.39,28.83 45.71,28.83
  Top 0.61: OUT_B.2 75.71,21.21 J2.2 | v69.84,29.14 67.93,29.14 67.22,29.86 62.46,29.86 D10.A 60.2,30.73 58.22,28.75 51.87,28.75 51.8,28.83 45.71,28.83 | v38.72,34.54 40.63,34.54 42.46,32.71 44.63,32.71 45.79,31.55 45.79,29.54 45.23,28.99 | 43.01,26.76 43.01,26.39 41.95,25.33 41.95,22.8 42.66,22.08 44.83,22.08 v45.39,21.52 48.25,21.52 | 48.25,21.52 K2_AB.P2 49.52,25.33 K4_B.5 | K4_B.6 48.25,21.52
  Bottom 0.457: v45.39,21.52 45.39,20.57 45.07,20.25 JP_LED1.1
  Bottom 0.61: ABC2.1 67.3,29.78 67.62,29.46 69.52,29.46 v69.84,29.14 69.84,24.38 J2.2 | D12.C 35.87,34.54 v38.72,34.54
B_NC  (via drill 0.35)
  Top 0.457: 27.93,36.77 27.93,38.99 27.61,39.3 26.03,39.3 24.12,41.21 24.12,43.12 13.96,43.12 12.25,41.4 12.25,39.78 11.1,38.64 J7.2 | 27.93,36.77 27.93,35.81 | v34.6,36.77 27.93,36.77
  Top 0.61: J2.1 70.16,20.89 R3.2 | K4_B.1 57.14,24.06 K2_AB.O2 v53.65,26.29 | D6.C v38.72,35.81 | D12.A 27.93,35.81
  Bottom 0.457: v38.72,35.81 36.3,35.81 36.23,35.88 35.49,35.88 v34.6,36.77
  Bottom 0.61: OUT_B.1 75.08,23.75 J2.1 | R3.2 60.95,26.61 K4_B.1 | D6.C 44.12,35.81 46.59,33.35 49.96,33.35 50.23,33.08 50.23,29.7 v53.65,26.29 | ABC.2 8.46,37.72 J7.2
B_NO
  Top 0.61: J2.3 R4.2
  Bottom 0.61: OUT_B.3 74.75,18.67 J2.3 | R4.2 66.35,18.67 K2_AB.S2 60.95,22.79 K4_B.10
C_CO  (via drill 0.35)
  Top 0.61: v68.57,30.73 65.95,33.35 57.44,33.35 55.16,35.63 55.16,37.04 54.41,37.79 53.89,37.79 v53.65,38.04
  Bottom 0.457: 50.31,41.37 50.47,41.53 | 68.57,32.32 67.3,32.32 ABC2.2
  Bottom 0.61: OUT_C.2 73.18,33.75 J3.2 71.43,32.32 68.57,32.32 v68.57,30.73 | v53.65,38.04 50.31,41.37 K3_C.6 | 50.47,41.53 50.79,41.84 K1_CD.P1 49.52,44.39 K3_C.5
C_NC
  Top 0.61: K1_CD.O1 57.14,43.12 K3_C.1 60.24,45.1 61.45,45.1 62.17,44.38 62.17,44.01 66.17,40.02 67.22,40.02 70.79,36.45 J3.1
  Bottom 0.61: OUT_C.1 75.08,36.45 J3.1 | K1_CD.O1 54.28,44.7 ABC3.2
C_NO
  Top 0.61: K3_C.10 62.46,37.79 63.3,37.79 63.57,37.53 63.57,37.33 69.52,31.37 J3.3
  Bottom 0.61: OUT_C.3 74.75,31.37 J3.3 | K3_C.10 59.68,41.84 K1_CD.S1
COM  (via drill 0.35)
  Top 0.457: 60.63,46.61 60.31,46.93 56.5,46.93 56.19,47.24
  Top 0.508: 25.39,44.44 26.12,44.44 26.14,44.41 27.59,44.41 v27.93,44.07
  Top 0.61: v52.06,53.59 v54.28,51.37 54.65,51 54.65,48.78 56.19,47.24 | v62.85,54.55 v62.85,56.45 | v63.17,45.97 61.27,45.97 60.63,46.61 | 25.39,44.44 12.83,44.44 12.64,44.25 ABC.4 7.99,45.66 5.67,47.98 5.67,57.82 7.54,59.69 10.14,59.69 12.69,62.24 15.94,62.24 v16.18,62.48 | v30.15,39.3 31.74,39.3 32.38,38.67 v33.64,38.67
  Bottom 0.457: v52.06,53.59 53.33,54.86 53.33,57.09 53.65,57.4 54.6,57.4 ABC4.1 | v62.85,56.45 62.85,61.21 62.22,61.85 NWS2.2 | v30.15,39.3 30.47,39.62 30.47,44.39 28.25,44.39 v27.93,44.07 | WS4.1 16.5,62.8 v16.18,62.48
  Bottom 0.61: ABC3.1 54.28,48.2 | 54.28,48.2 v54.28,51.37 | v63.17,45.97 63.17,54.23 v62.85,54.55 | ABC.4 9.44,42.8 J7.4 | v33.64,38.67 33.76,38.55 33.76,32.55 35.37,30.94 35.37,19.46 34.86,18.95 34.86,10.2 38.54,6.53 40.18,6.53 42.46,8.8 42.46,9.59 42.73,9.85 46.15,9.85 46.38,9.62 48.47,9.62 48.7,9.85 52.14,9.85 54.48,12.2 54.48,25.94 54.68,26.13 54.68,38.19 53.01,39.85 53.01,46.93 54.28,48.2
CTRL_H_OB2  (via drill 0.35)
  Top 0.457: v47.3,65.66 46.66,65.66 46.34,65.34 42.22,65.34 39.04,62.16 32.69,62.16 32.38,62.48 26.34,62.48 21.58,57.72 21.58,55.82 K_RES_H.9
  Bottom 0.457: v47.3,65.66 48.25,66.61 RES_H.2
D_CO  (via drill 0.35)
  Top 0.457: 67.3,52.64 66.03,52.64
  Top 0.61: J4.2 68.01,51.61 68.01,51.93 67.3,52.64 | 66.03,52.64 62.61,52.64 60.63,54.62 51.91,54.62 50.56,53.28 K4_D.5 | K4_D.6 49.2,47.88 v46.03,47.88
  Bottom 0.457: v46.03,47.88 45.07,46.93 JP_LED2.1 | 65.71,37.08 66.03,37.4 67.3,37.4
  Bottom 0.61: OUT_D.2 73.18,46.45 J4.2 73.02,46.04 71.62,44.65 71.62,41.72 67.3,37.4 | ABC1.2 64.76,36.13 65.71,37.08 | K4_D.5 50.79,52.01 K2_CD.P2 50.79,49.47 K4_D.6
D_NC
  Top 0.457: 56.5,50.73 K2_CD.O2
  Top 0.61: R6.2 62.17,50.79 62.17,52 61.45,52.72 60.24,52.72 K4_D.1 59.04,53.28 56.5,50.73
  Bottom 0.61: OUT_D.1 75.08,49.15 J4.1 70.16,46.29 R6.2 | K2_CD.O2 55.75,50.85 55.75,53.62 54.6,54.77 ABC4.2
D_NO
  Top 0.61: J4.3 R5.2 66.26,44.07 62.72,47.61 60.26,47.61 K4_D.10 59.68,49.47 K2_CD.S2
  Bottom 0.61: OUT_D.3 74.75,44.07 J4.3
DI_WS1  (via drill 0.35)
  Top 0.457: v20.63,16.45 22.85,14.22 U2R.6
  Bottom 0.457: v20.63,16.45 18.41,16.45 18.41,17.71 U3H.6 18.09,18.03 17.77,18.35 17.77,19.94 16.5,21.21 13.32,21.21 13.32,16.13 11.42,18.03 11.42,18.67 11.74,18.98 11.74,21.52 9.2,21.52 7.93,20.25 CON1.2
  Bottom 0.61: SV4.2 16.32,3.13 16.32,8.01 13.32,11.01 13.32,16.13
DO1_DI2  (via drill 0.35)
  Top 0.457: v19.04,27.88 U4R.6
  Bottom 0.203: 21.58,15.81 18.36,15.81 17.01,17.16 U3H.5
  Bottom 0.457: SINGLE.2 18.41,38.04 U5H.6 18.41,35.5 18.72,35.18 18.72,34.86 21.9,31.68 U4R.6 | U2R.5 22.85,11.68 21.58,12.95 21.58,15.81 21.58,18.98 19.04,21.52 v19.04,27.88
DO2_DI3  (via drill 0.35)
  Top 0.457: v17.45,39.3 18.41,39.3 22.21,35.5 23.48,35.5 24.12,34.86 24.12,30.41 U4R.5 | v23.17,69.47 v23.17,72.01 | v16.82,58.67 20.63,58.67 v23.48,61.53
  Bottom 0.457: U5H.5 17.14,38.04 SINGLE.1 17.45,38.04 v17.45,39.3 16.5,40.26 16.5,47.45 15.23,48.72 15.23,53.28 15.76,53.28 16.82,54.34 v16.82,58.67 | NO_OPTW1.2 24.12,78.67 24.12,78.04 22.85,76.77 22.85,72.33 v23.17,72.01 | v23.17,69.47 22.85,69.15 22.85,64.7 23.8,63.75 23.8,62.16 23.96,62.01 | 23.96,62.01 24.44,61.53 U6H.6 25.39,61.53 26.34,62.48 26.34,63.12 U5R.6 | 23.96,62.01 v23.48,61.53
DO3_DI4  (via drill 0.35)
  Top 0.457: U5R.5 31.11,65.98 29.2,64.07 25.39,64.07 | v22.21,64.07 25.39,64.07 | v26.79,71.56 26.79,70.27 25.52,68.99 25.52,64.2 25.39,64.07
  Bottom 0.457: NO_OPTW2.2 29.2,78.67 | 29.2,78.67 NO_OPTW1.1 | 29.2,78.67 U7R.6 26.66,73.59 26.66,72.64 25.71,71.69 U8H.6 26.66,71.69 v26.79,71.56 | U6H.5 22.21,60.26 v22.21,64.07
DO4_NEXT_TERM  (via drill 0.35)
  Top 0.152: v17.45,72.33 22.53,72.33 24.44,74.23 30.15,74.23 30.15,75.5 30.79,76.14 U7R.5
  Bottom 0.152: 31.11,78.67 31.11,75.82 U7R.5 | 31.11,78.67 NO_OPTW2.1 31.11,78.67 | 31.11,78.67 32.06,79.63 34.6,79.63 34.6,78.67 TERM.2 | v17.45,72.33 17.45,78.67 SV3.2
  Bottom 0.254: U7R.5 31.37,75.77 30.48,75.77 27.98,73.27 27.98,71.81 26.59,70.42 U8H.5
DO_RETURN  (via drill 0.35)
  Top 0.152: v32.69,77.09 32.38,77.09 32.06,77.41 27.93,77.41 27.93,75.82 26.66,74.55 v21.9,74.55
  Top 0.457: v21.58,25.02 21.26,25.02 20.95,25.33 12.37,25.33 11.1,24.06 9.2,24.06 7.93,22.79 CON1.4 7.93,23.11 v5.71,25.33
  Top 0.61: SV3.4 17.73,73.96 14.4,73.96 12.19,71.75 v11.42,71.75 | SV4.4 24.79,3.94 v24.79,4.98
  Bottom 0.152: v32.69,77.09 33.01,77.41 33.64,77.41 33.64,78.67 TERM.1
  Bottom 0.203: SV3.4 22.69,77.66 21.9,76.87 v21.9,74.55
  Bottom 0.457: v21.58,25.02 21.58,23.75 24.75,20.57 24.73,20.55 24.73,9.84 24.79,9.78 v24.79,4.98 | v5.71,25.33 5.71,72.01 8.88,72.01 9.13,71.75 v11.42,71.75
E_CO  (via drill 0.35)
  Top 0.457: 11.42,18.35 6.66,13.59 6.34,13.27 6.34,9.46 6.97,8.83 10.79,8.83 14.91,4.7 21.58,4.7 | 26.63,4.7 26.66,4.7
  Top 0.61: J5.2 75.71,59.31 OUT_E.2 75.87,58.46 78.13,56.21 78.13,16.98 78.11,16.98 76.69,15.56 74.04,15.56 69.52,11.05 v69.52,9.46 | v52.06,72.96 52.33,72.69 55.2,72.69 56.15,71.74 60.95,71.74 61.53,71.16 64.09,71.16 64.16,71.23 67.12,71.23 68.73,69.62 68.73,69.51 69.84,68.41 v69.84,67.25 | 6.66,13.59 6.26,13.19 6.26,9.54 7.05,8.75 10.75,8.75 14.77,4.74 21.54,4.74 | 6.34,13.27 11.42,18.35 v12.37,18.35 | 21.58,4.7 23.33,4.7 24.45,5.81 25.14,5.81 26.25,4.7 26.63,4.7 | 26.66,4.7 v33.01,4.7
  Bottom 0.61: v52.06,72.96 52.06,67.26 52.01,67.21 52.01,64.32 50.44,62.75 50.1,62.75 K3_E.5 49.52,60.9 K1_EF.P1 49.52,58.36 K3_E.6 | v12.37,18.35 12.37,18.65 12.42,18.7 12.42,33.52 12.32,33.62 12.32,39.04 J7.3 8.48,40.26 ABC.3 | v69.52,9.46 68.81,8.75 63.58,8.75 59.61,4.77 43.62,4.77 42.46,3.61 42.46,2.83 41.07,1.45 37.65,1.45 37.28,1.82 37.28,3.19 35.77,4.7 v33.01,4.7 | v69.84,67.25 69.84,62.48 J5.2
E_NC  (via drill 0.35)
  Top 0.61: K3_E.1 64.02,62.16 66.08,60.11 67.3,60.11 67.33,60.14 69.09,60.14 70.79,61.85 J5.1 | v58.73,59.62 K1_EF.O1
  Bottom 0.457: WS1.2 NWS2.1 62.22,62.8 59.68,62.8 K3_E.1
  Bottom 0.61: OUT_E.1 75.08,61.85 J5.1 | K3_E.1 59.68,60.58 v58.73,59.62 | K1_EF.O1 54.92,60.58 WS3.2
E_NO  (via drill 0.35)
  Top 0.457: v58.41,65.66 58.41,64.07 59.04,63.44 60.56,63.44 60.63,63.36 | J5.3 72.38,57.4 66.03,57.4 65.76,57.67 v65.66,57.67 64.23,59.1 64.16,59.17 63.79,59.54 63.79,59.62
  Top 0.61: 63.79,59.62 K1_EF.S1 | v65.39,62.48 64.78,62.48 63.9,63.36 60.63,63.36
  Bottom 0.457: 58.57,65.82 v58.41,65.66 | 67.3,57.4 66.03,57.4 65.76,57.67 v65.66,57.67 65.13,58.2
  Bottom 0.61: OUT_E.3 74.75,56.77 J5.3 72.38,57.4 67.3,57.4 | v65.39,62.48 65.39,62.27 65.13,62.01 65.13,58.2 | WS2.2 59.36,66.61 58.57,65.82 | K3_E.10 59.68,58.36 K1_EF.S1
F_CO  (via drill 0.35)
  Top 0.457: 51.11,73.28 v50.79,72.96 | v38.09,78.67 34.28,78.67 24.75,78.67 19.36,73.28 16.5,73.28 16.16,72.94 14.34,72.94 12.4,70.99 v10.21,70.99 | v13.96,41.84 12.86,40.74 12.86,39.47 12.25,38.86 12.25,37.24 11.1,36.1 J7.1
  Top 0.61: OUT_F.2 73.18,73.12 J6.2 71.58,71.84 71.58,66.45 70.72,65.58 66.11,65.58 65.32,66.37 65.32,67.96 v64.76,68.52 | v59.04,73.59 53.96,73.59 53.89,73.52 52.68,73.52 52.41,73.8 51.62,73.8 51.11,73.28 | K4_F.6 49.2,64.39 v46.03,64.39
  Bottom 0.356: 10.12,55.82 10.12,55.63 10.89,54.86 11.95,54.86 13.96,52.85 13.96,52.01
  Bottom 0.406: v10.21,70.99 10.21,69.45 10.12,69.37 10.12,63.22 10.15,63.19 10.15,56.69 10.12,56.67 10.12,55.82
  Bottom 0.457: 13.96,52.01 v13.96,41.84 | v38.09,78.67 49.52,78.67 49.52,76.77 50.15,76.14 52.06,76.14 52.06,74.23 v50.79,72.96
  Bottom 0.61: NWS1.1 79.05,73.59 78.57,73.12 OUT_F.2 | v50.79,72.96 50.79,71.06 K4_F.5 49.52,68.52 K2_EF.P2 49.52,65.98 K4_F.6 | JP_LED3.1 45.71,63.44 46.03,63.75 v46.03,64.39 | ABC.1 9.42,35.18 J7.1 | v64.76,68.52 59.68,73.59 v59.04,73.59
F_NC  (via drill 0.35)
  Top 0.61: v64.76,69.78 K4_F.1
  Bottom 0.457: K4_F.1 59.68,68.83
  Bottom 0.61: WS2.1 59.36,68.52 59.68,68.83 58.09,68.83 57.7,68.44 57.06,68.44 K2_EF.O2 55.55,67.56 54.28,67.56 53.96,67.25 ABC5.1 | NWS1.2 79.05,76.14 78.57,76.62 OUT_F.1 75.08,75.82 J6.1 70.16,72.96 R8.2 68.57,71.06 66.03,71.06 v64.76,69.78
F_NO
  Top 0.457: R7.2 60.31,64.07 K4_F.10
  Top 0.61: K4_F.10 60.26,64.12 64.73,64.12 64.78,64.07 R7.2 70.33,64.07 OUT_F.3
  Bottom 0.61: OUT_F.3 74.75,70.74 J6.3 | K4_F.10 59.68,65.51 60.45,66.29 60.45,66.75 K2_EF.S2 62.22,65.98 WS1.1
G_COM  (via drill 0.35)
  Top 0.457: OUT_G.2 7.93,66.29 J8.2 v14.91,66.29 | K_RES_G.5 K_RES_G.6
  Bottom 0.457: K_RES_G.5 15.23,65.98 v14.91,66.29 16.18,66.29 16.5,65.98 WS4.2
G_NC  (via drill 0.35)
  Top 0.457: v53.01,62.8 50.79,62.8 50.15,63.44 v41.58,63.44 | v41.27,65.66 37.77,65.66 36.82,64.7 30.79,64.7 29.2,63.12 16.82,63.12 16.34,63.59 | 16.34,63.59 16.18,63.75 J8.1 8.72,63.75 OUT_G.1 | K_RES_G.1 15.23,70.42 16.5,69.15 16.5,63.75 16.34,63.59
  Bottom 0.457: v41.58,63.44 41.27,63.75 v41.27,65.66
  Bottom 0.61: WS3.1 54.92,63.42 54.91,63.43 53.64,63.43 v53.01,62.8
G_NO
  Top 0.457: K_RES_G.10 17.14,71.06 15.86,72.33 14.59,72.33 11.9,69.63 | 11.9,69.63 11.42,69.15 J8.3 | OUT_G.3 7.93,69.78 11.74,69.78 11.9,69.63
GND  (via drill 0.35)
  Top 0.457: LED1.K 66.35,11.37 65.08,12.63 65.08,26.92 LED2.K | LED5.K LED4.K | C3R1.2 37.14,71.06 38.09,72.01 54.92,72.01 55.87,71.06 60.21,71.06 60.79,70.47 64.37,70.47 64.45,70.54 65.59,70.54 LED6.K | LED3.K 66.03,36.13 v64.44,37.72 | LED7.K 9.52,12.63 11.1,14.22 12.69,14.22 12.85,14.06 13.01,14.22
  Top 1.27: C2.2 18.94,40.47 16.74,40.47 13.68,37.41 13.68,31.04 15.23,29.49 U4R.4 12.44,26.35 11.95,26.35 10.94,25.33 CON1.5 | U2R.4 12.85,13.97 12.85,14.06 | 13.01,14.22 13.54,14.75 13.54,21.95 12.69,22.79 CON1.3
  Bottom 0.457: LED3.K 66.03,35.5 66.03,29.14 LED2.K | 64.6,57.24 66.67,55.18 LED4.K | 64.6,57.24 64.44,57.4 64.44,66.5 66.67,68.72 LED6.K | 31.58,59.15 31.74,58.99 U5R.4 31.74,50.73 | 31.58,59.15 30.47,60.26 U6H.4 | 31.58,59.15 31.74,59.31 33.96,59.31 C3H.2 33.96,60.9 C3R.2 37.77,62.16 37.77,66.29 34.28,69.78 | 31.58,69.63 31.74,69.47 U7R.4 | 31.58,69.63 30.79,70.42 U8H.4 | C3R1.2 34.28,71.06 C3H1.2 34.28,69.78 | 34.28,69.78 31.74,69.78 31.58,69.63 | v64.44,37.72 64.44,57.09 64.6,57.24 | IC2.8 30.47,36.77 | U3H.4 16.82,12.63 15.55,11.37 U2R.4 | C1R.2 17.77,6.28 17.77,8.83 C1H.2 17.45,9.14 | U5H.4 17.14,30.1 15.23,30.1 U4R.4 17.45,26.92 17.45,26.61 C2H.2 17.77,26.61 C2R.2 C4.2 | 30.83,12.63 30.81,12.62 IC1.8 | 31.74,50.73 31.74,41.84 C5.2 32.38,39.94 32.38,33.59 | C3.2 31.74,50.73 | C7.2 30.83,18.98 | C6.2 30.83,25.33 | C9.2 18.63,53.28
  Bottom 0.508: 30.83,28.23 29.9,29.16 25.38,29.16 25.01,29.53 | 30.47,36.77 30.47,34.23 31.11,33.59 32.38,33.59
  Bottom 1.016: 22.57,38.31 22.7,38.19 23.44,38.19 24.27,37.35 24.27,33.14 24.88,32.53 24.88,29.65 25.01,29.53
  Bottom 1.27: SV3.3 20.15,73.27 18.63,71.75 18.63,53.28 18.63,43.52 C2.2 20.31,40.58 22.57,38.31 | 32.38,33.59 32.38,29.78 30.83,28.23 30.83,25.33 30.83,18.98 30.83,12.63 30.83,7.91 C1.2 29.2,6.28 C8.2 26.66,5.13 24.92,3.39 22.05,3.39 21.53,2.87 21.18,2.87 SV4.3 17.78,4.21 C1R.2 17.45,6.35 17.45,9.14 17.45,9.37 U2R.4 | CON1.5 CON1.3
  pour Bottom: 0.62,79.95 83.81,79.95 83.81,1.21 0.62,1.21
H_COM  (via drill 0.35)
  Top 0.457: J9.2 7.93,53.59 OUT_H.2 | K_RES_H.6 15.86,46.93 | 15.86,46.93 v13.01,49.78 | 15.86,46.93 K_RES_H.5
  Bottom 0.457: J9.2 13.01,52.01 v13.01,49.78
H_NC
  Top 0.457: K_RES_H.1 15.23,56.45 13.01,54.23 13.01,52.64 J9.1
  Bottom 0.457: J9.1 11.42,50.42 7.93,50.42 OUT_H.1
H_NO
  Top 0.457: K_RES_H.10 17.14,57.09 15.86,58.36 13.64,58.36 12.21,56.93 | J9.3 12.21,56.93 | OUT_H.3 7.93,57.09 12.05,57.09 12.21,56.93
IB1
  Top 0.457: IC1.6 RN1.3 25.39,16.45 25.39,12.32 23.17,10.1 22.53,10.1 18.72,13.91 15.55,13.91 U2R.3
  Bottom 0.305: C8.1 27.93,10.1 27.93,16.45 29.19,17.7 IC1.6
  Bottom 0.457: U3H.3 18.09,12.95 17.77,13.27 17.77,13.91 17.45,14.22 15.55,14.22 U2R.3
IB1_2
  Top 0.152: IC1.7 30.48,16.45 35.56,16.45 IC1.11
  Top 0.457: RN1.2 IC1.7
IB2  (via drill 0.35)
  Top 0.457: v13.01,43.43 13.32,43.75 26.03,43.75 RN2.3 IC2.6 C5.1
  Bottom 0.457: U5H.3 18.41,30.41 18.09,30.73 18.09,31.05 17.45,31.68 U4R.3 13.01,33.91 v13.01,43.43
IB2_2
  Top 0.457: RN2.2 IC2.7 30.47,41.84 33.46,41.84 34.94,43.32 34.94,46.32 35.55,46.93 37.45,46.93 38.09,46.29 38.09,45.02 36.82,43.75 IC2.11
IB3  (via drill 0.35)
  Top 0.457: v39.68,57.4 39.36,57.4 39.04,57.09 30.47,57.09 U5R.3
  Bottom 0.457: U6H.3 28.88,61.53 28.88,58.67 U5R.3 | OPT_LED.4 49.52,73.59 41.58,73.59 41.58,73.91 40.95,74.55 39.68,74.55 v39.68,57.4
IB4
  Top 0.457: OPT_LED.8 43.17,74.87 40.95,72.64 37.77,72.64 37.45,72.33 33.01,72.33 U7R.3
  Bottom 0.254: U8H.3 29.52,71.69 29.2,71.37 U7R.3
IG1  (via drill 0.35)
  Top 0.457: IC1.4 RN1.5 24.15,20.29 19.9,20.29 19.24,19.62 v16.82,19.62 | IC1.4 | C7.1 30.47,21.52 IC1.4
  Bottom 0.203: v16.82,19.62 16.34,19.14 U2R.1 15.29,18.21 18.05,15.46 18.21,15.46 18.21,15.45 20.03,15.45 20.82,14.67 U3H.1
IG1_2
  Top 0.457: RN1.4 IC1.5 29.21,20.25 34.6,20.25 36.82,22.48 IC1.13
IG2  (via drill 0.35)
  Top 0.457: IC2.4 RN2.5 23.48,48.2 20.63,45.34 v14.91,45.34 | v18.88,32.79 18.88,30.25 C4.1
  Bottom 0.457: v14.91,45.34 14.91,37.08 U4R.1 15.23,35.84 16.37,34.7 16.37,34.35 17.14,33.59 18.08,33.59 v18.88,32.79 20.36,31.31 20.36,30.94 U5H.1
IG2_2
  Top 0.457: RN2.4 IC2.5 31.74,48.2 IC2.13
IG3  (via drill 0.35)
  Top 0.457: v60,38.99 42.85,38.99 40.63,36.77 v37.77,36.77 | v34.6,58.04 v31.74,60.9 29.2,60.9 27.8,59.5 27.8,57.88 27.13,57.21 26.19,57.21 25.04,58.36 U5R.1
  Bottom 0.457: OPT_LED.3 52.06,78.67 54.6,78.67 54.6,76.77 63.81,67.56 63.81,56.13 63.17,55.5 61.9,55.5 61.9,52.32 62.22,52.01 62.22,41.21 v60,38.99 | v31.74,60.9 31.74,63.44 31.11,64.07 U6H.1
  Bottom 0.61: v37.77,36.77 37.38,36.77 37.36,36.74 36.28,36.74 34.6,38.43 v34.6,58.04
IG4  (via drill 0.35)
  Top 0.457: OPT_LED.7 39.68,77.41 37.14,74.87 31.39,74.87 31.15,75.11 v30.86,75.11
  Bottom 0.254: U8H.1 29.52,74.23 28.39,73.1 28.39,70.42 27.52,69.56 26.23,69.56 25.19,68.52 U7R.1
  Bottom 0.457: U8H.1 30.86,74.56 v30.86,75.11
IR1  (via drill 0.35)
  Top 0.203: U2R.2 19.89,16.6 20.91,17.62 24.03,17.62 25.39,18.98 v25.49,18.98
  Top 0.457: RN1.7 IC1.2 | IC1.2 | C6.1 IC1.2
  Bottom 0.203: U3H.2 19.55,13.4 18.24,14.71 16.82,14.71 15.29,16.23 U2R.2 | v25.49,18.98 25.37,19.11 25.37,20.68
  Bottom 0.457: IC1.2 29.2,27.56 27.93,26.29 27.93,22.34 27.16,21.58 26.26,21.58 25.37,20.68
IR1_2
  Top 0.457: RN1.6 IC1.3 30.48,26.61 35.52,26.61 36.13,27.21 36.17,27.21 IC1.15
IR2  (via drill 0.35)
  Top 0.457: U4R.2 17.14,34.86 v19.36,37.08 | v16.5,51.69 25.07,51.69 RN2.7 IC2.2 C3.1
  Bottom 0.457: RN2.7 26.66,52.96 24.75,52.96 RES_G2.2 | v16.5,51.69 16.5,48.31 17.11,47.7 17.11,41.03 19.36,38.78 v19.36,37.08 | U5H.2 19.09,30.94 19.09,31.31 17.44,32.96 16.5,32.96 U4R.2
IR2_2
  Top 0.457: RN2.6 IC2.3 30.47,52.01 34.28,52.01 35.55,53.28 IC2.15
IR3
  Top 0.457: RN1.8 IC1.1
  Bottom 0.457: RES_G1.2 24.75,54.55 | 24.75,54.55 RES_G2.1 | 24.75,54.55 24.81,54.49 27.16,54.49 27.88,53.78 27.88,52.77 27.16,52.06 26.26,52.06 25.44,51.24 25.44,42.61 26.26,41.79 27.16,41.79 27.98,40.98 27.98,36.51 29.58,34.91 29.58,33.54 29.2,33.16 IC1.1
IR3_2  (via drill 0.35)
  Top 0.457: v51.11,64.7 v53.01,64.7 | v47.93,62.48 40.31,62.48 37.45,59.62 34.28,59.62 32.06,61.85 27.93,61.85 26.66,60.58 U5R.2
  Bottom 0.457: OPT_LED.2 53.01,74.55 53.01,67.25 52.7,66.93 52.7,65.02 v53.01,64.7 | v51.11,64.7 50.79,64.39 50.79,64.07 50.15,63.44 47.93,63.44 v47.93,62.48 | C9.1 22.85,57.09 24.75,57.09 | 24.75,57.09 25.39,57.09 U5R.2 26.66,61.53 27.93,62.8 U6H.2 | RES_G1.1 24.75,57.09
IR3_3  (via drill 0.35)
  Top 0.457: v31.42,34.86 35.87,30.41 IC1.16 | IC2.1 RN2.8
  Bottom 0.457: v31.42,34.86 31.11,35.18 31.11,44.61 30.47,45.25 30.47,54.55 IC2.1
IR4
  Bottom 0.254: 38.09,76.14 37.81,76.41 37.81,76.55 37.23,77.13 33.87,77.13 33.29,76.55 33.29,75.49 31.45,73.65 31.22,73.65 U8H.2 29.52,72.96 28.79,72.24 28.79,69.56 28.77,69.56 27.73,68.52 U7R.2
  Bottom 0.457: OPT_LED.6 46.98,76.14 38.09,76.14
LED2
  Top 0.457: R3.1 LED2.A
LED3
  Bottom 0.457: R5.1 LED3.A
LED4
  Top 0.457: R6.1 LED4.A
LED_1
  Top 0.457: LED1.A 66.98,13.27 R4.1
LED_5
  Bottom 0.457: R7.1 LED5.A
LED_6
  Bottom 0.61: LED6.A 66.98,66.93 R8.1
LED_7
  Top 0.457: R9.2 LED7.A
N$6
  Bottom 0.457: 6=5V.1 6.97,16.45 6.34,17.08 6.34,23.43 7.61,24.7 7.61,25.33 CON1.6
N$16
  Top 0.61: D1.A 43.8,8.51 D2.C
N$19
  Top 0.61: D2.A D3.C
N$21
  Top 0.61: D4.C D3.A
N$23
  Top 0.61: D4.A D5.C
N$24
  Bottom 0.61: D7.A 52.06,36.45 D8.C
N$25
  Top 0.61: D9.C 56.5,30.73 D8.A
N$26
  Top 0.61: D10.C 57.77,35.81 D9.A
N$27
  Bottom 0.61: D7.C 47.61,30.73 D6.A
N$42
  Top 0.457: LED8.K 42.22,68.83 43.17,69.78 R12.1
N$43
  Top 0.457: LED9.K 41.9,58.36 43.17,57.09 R13.1
N$44
  Bottom 0.457: LED10.K 44.44,53.91 R14.1
N$45
  Bottom 0.457: LED11.K 44.44,39.94 R15.1
N$46
  Bottom 0.457: LED12.K 44.76,27.88 R16.1
N$47
  Top 0.457: LED13.K 46.03,12.63 R17.1
OB1
  Top 0.457: 45.07,48.83 K2_CD.16 | 45.07,48.83 46.34,48.83 46.98,49.47 R14.2 | K3_C.2 51.42,45.66 50.15,46.93 45.71,46.93 45.07,47.56 45.07,48.83
  Bottom 0.457: K2_CD.16 40.63,48.2 40.63,39.3 41.9,38.04 41.9,29.35 40.95,28.4 40.95,27.24 40.31,26.61 40.31,20.89 40.95,20.25 40.95,11.37 39.04,11.37 38.41,12 38.41,13.27 36.82,14.86 IC1.10
OB2  (via drill 0.35)
  Top 0.457: IC2.10 36.82,41.21 40.31,44.7 v40.31,49.78 | v55.55,74.55 53.96,76.14 43.17,76.14 v40.63,73.59 | v40.63,70.42 39.68,69.47 39.68,67.56 v40.63,66.61
  Bottom 0.457: K1_EF.15 45.71,67.56 48.25,67.56 RES_H.1 | v40.31,49.78 40.63,50.1 40.63,54.55 41.58,55.5 46.98,55.5 R13.2 46.98,64.7 46.34,65.34 46.34,66.61 K1_EF.15 | K4_F.2 55.55,71.37 v55.55,74.55 | v40.63,70.42 v40.63,73.59 | v40.63,66.61 40.31,66.29 40.31,63.44 41.27,62.48 42.53,62.48 42.53,63.75 45.71,66.93 K1_EF.15
OG1
  Top 0.457: K4_B.2 57.77,26.61 59.04,27.88 60.31,27.88 62.22,25.97 62.22,14.54 60.31,12.63 48.57,12.63 R17.2
  Bottom 0.406: MONO3.2 48.25,25.02 47.04,25.02 45.96,23.94
  Bottom 0.457: 46.34,23.75 45.71,23.75 K1_AB.15 45.96,23.94 46.34,23.75 | 44.44,10.73 46.98,10.73 R17.2 | 44.44,10.73 36.82,10.73 35.55,12 35.55,18.67 36.82,19.94 IC1.12 | 46.34,23.75 46.34,19.62 44.44,17.71 44.44,10.73
OG2  (via drill 0.35)
  Top 0.457: 56.35,62.96 52.06,67.25 52.06,69.15 50.15,71.06 48.25,71.06 R12.2 | 56.35,62.96 K3_E.2 | v47.3,20.57 43.17,20.57 40.95,22.79 40.95,31.25 37.97,34.23 37.97,34.35 35.55,36.77 35.55,44.39 IC2.12 | 56.35,62.96 52.06,58.67 52.06,57.72 49.52,55.18 38.41,55.18 v38.09,54.86
  Bottom 0.406: MONO3.1 48.25,22.79 47.3,21.84 47.3,21.52
  Bottom 0.457: K1_EF.16 42.85,67.56 42.85,70.1 44.12,71.37 46.98,71.37 R12.2 | v47.3,20.57 47.3,21.52 | v38.09,54.86 38.09,46.93 IC2.12
OR1  (via drill 0.35)
  Top 0.457: IC1.14 36.82,25.02 40.63,21.21 v41.27,21.21 42.85,19.62 48.25,19.62 48.88,20.25 56.19,20.25 56.35,20.41 | K3_A.2 57.14,19.62 56.35,20.41 | 56.35,20.41 52.06,24.7 52.06,25.97 50.15,27.88 48.57,27.88 R16.2
  Bottom 0.457: K1_AB.16 41.27,22.16 v41.27,21.21
OR2  (via drill 0.35)
  Top 0.457: IC2.14 40.63,50.73 46.98,44.39 R15.2 | v54.92,53.28 K4_D.2
  Bottom 0.457: K1_CD.15 46.98,49.47 46.98,46.93 | R15.2 46.98,46.93 | v54.92,53.28 52.06,50.42 52.06,48.83 50.15,46.93 46.98,46.93
OR3  (via drill 0.35)
  Top 0.457: IC2.16 31.42,55.82 30.31,54.7 30.15,54.55 v22.18,54.55
  Bottom 0.457: K_RES_G.9 20.31,64.7 21.58,63.44 21.58,55.15 v22.18,54.55
PWR_WS1  (via drill 0.35)
  Top 0.457: v19.99,19.3 22.85,19.3 U2R.8
  Bottom 0.457: v19.99,19.3 20.31,18.98 20.31,18.35 20.63,18.03 U3H.8 | C1R.1 20.31,6.28 20.31,8.83 C1H.1 20.63,8.83 R1.2 24.12,10.1 24.12,18.03 23.17,18.98 U2R.8
PWR_WS2
  Bottom 0.457: U4R.8 22.85,35.81 22.41,35.37 21.71,35.37 | C2R.1 20.31,26.61 C2H.1 R2.2 22.85,27.53 21.71,28.67 21.71,29.62 22.63,30.54 23.32,30.54 23.99,31.21 23.99,32.16 23.07,33.08 22.38,33.08 21.71,33.75 21.71,35.37 | U5H.8 21.52,35.55 21.71,35.37
PWR_WS3
  Bottom 0.457: U6H.8 24.75,64.07 24.12,64.7 U5R.8 25.39,67.25 33.96,67.25 R10.2 C3H.1 33.96,63.44 C3R.1
PWR_WS4
  Top 0.457: U7R.8 24.75,76.14 26.66,78.04 33.01,78.04 34.28,76.77 R11.2
  Bottom 0.457: U7R.8 24.12,75.18 25.07,74.23 U8H.8 | R11.2 C3H1.1 34.28,73.59 C3R1.1

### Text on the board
Top: Top
Bottom: Bot
tNames: wiki.mobaledlib.de | NC | NO | + | NO | + | NC | NC | + | NO | + | + | NO | NC | + | NC | Com | by Hardi | NO | Halt | + | NC | + | WS2811 Relais | VA | NO | NC | + | + | NO | + | + | NC | + | NO | by Hardi
bNames: => | <= | +5V | GND | wiki.mobaledlib.de | by Hardi | MobaLedLib@gmx.de | WS2811 Relais | <= | +5V | => | GND

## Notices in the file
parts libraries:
SparkFun-Retired: Licensing:Creative Commons ShareAlike 4.0 International - https://creativecommons.org/licenses/by-sa/4.0
